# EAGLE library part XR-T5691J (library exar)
T1 receive BUFFER
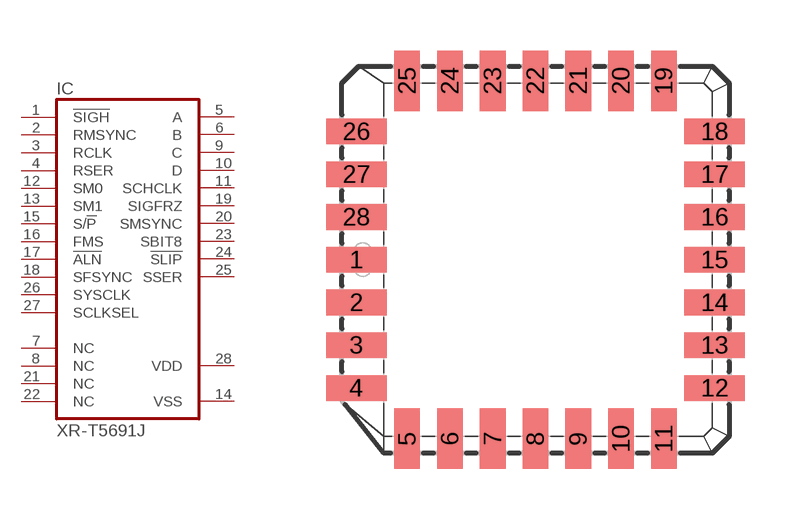
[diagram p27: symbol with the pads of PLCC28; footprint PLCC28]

Designator prefix IC

## XR-T5691J (OC_FARNELL: unknown; OC_NEWARK: unknown)  [PLCC28]
1  !SIGH  in
2  RMSYNC  in
3  RCLK  in
4  RSER  in
5  A  out
6  B  out
7  NC  nc
8  NC  nc
9  C  out
10  D  out
11  SCHCLK  out
12  SM0  in
13  SM1  in
14  VSS  pwr
15  S/!P  in
16  FMS  in
17  !ALN  in
18  SFSYNC  in
19  SIGFRZ  out
20  SMSYNC  out
21  NC  nc
22  NC  nc
23  SBIT8  out
24  !SLIP  out
25  SSER  out
26  SYSCLK  in
27  SCLKSEL  in
28  VDD  pwr

## Footprint PLCC28 (pad centres in mm)
Plastic Leaded Chip Carrier
smd 1.8 x 0.76: 1 -5.32,0; 2 -5.32,-1.27; 3 -5.32,-2.54; 4 -5.32,-3.81; 12 5.32,-3.81; 13 5.32,-2.54; 14 5.32,-1.27; 15 5.32,0; 16 5.32,1.27; 17 5.32,2.54; 18 5.32,3.81; 26 -5.32,3.81; 27 -5.32,2.54; 28 -5.32,1.27
smd 0.76 x 1.8: 5 -3.81,-5.32; 6 -2.54,-5.32; 7 -1.27,-5.32; 8 0,-5.32; 9 1.27,-5.32; 10 2.54,-5.32; 11 3.81,-5.32; 19 3.81,5.32; 20 2.54,5.32; 21 1.27,5.32; 22 0,5.32; 23 -1.27,5.32; 24 -2.54,5.32; 25 -3.81,5.32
